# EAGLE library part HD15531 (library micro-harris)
MICROCONTROLLER/MEMORY DEVICE
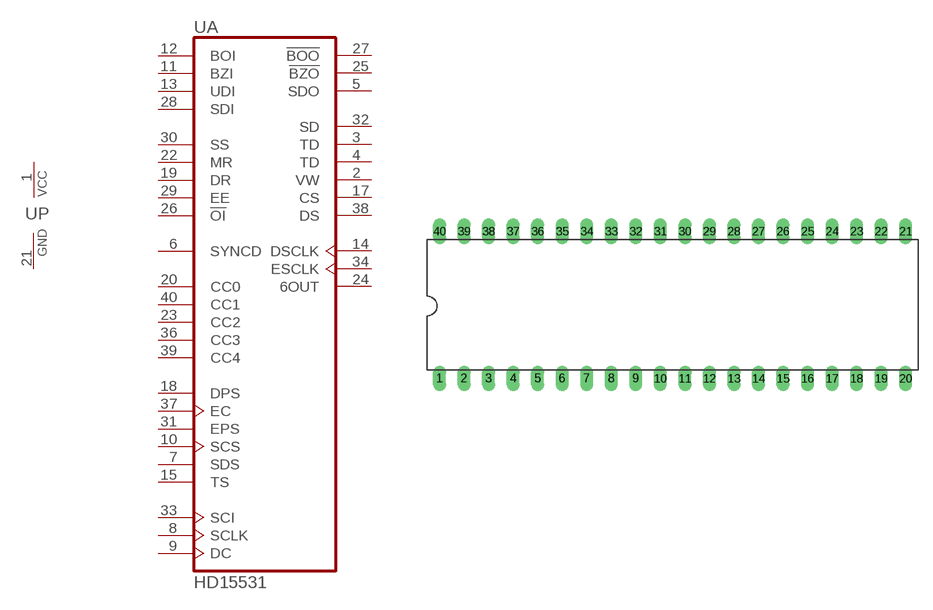
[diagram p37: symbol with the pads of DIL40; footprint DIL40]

Designator prefix U; gates A=HD15531 P=PWRN

## HD15531 (OC_FARNELL: unknown; OC_NEWARK: unknown)  [DIL40]
1  P:VCC  pwr
2  A:VW  out
3  A:TD  out
4  A:TD  out
5  A:SDO  out
6  A:SYNCD  in
7  A:SDS  in
8  A:SCLK  in
9  A:DC  in
10  A:SCS  in
11  A:BZI  in
12  A:BOI  in
13  A:UDI  in
14  A:DSCLK  out
15  A:TS  in
17  A:CS  out
18  A:DPS  in
19  A:DR  in
20  A:CC0  in
21  P:GND  pwr
22  A:MR  in
23  A:CC2  in
24  A:6OUT  out
25  A:!BZO  out
26  A:!OI  in
27  A:!BOO  out
28  A:SDI  in
29  A:EE  in
30  A:SS  in
31  A:EPS  in
32  A:SD  out
33  A:SCI  in
34  A:ESCLK  out
36  A:CC3  in
37  A:EC  in
38  A:DS  out
39  A:CC4  in
40  A:CC1  in

## Footprint DIL40 (pad centres in mm)
Dual In Line Package
drill 0.813 long: 1 -24.13,-7.62; 2 -21.59,-7.62; 3 -19.05,-7.62; 4 -16.51,-7.62; 5 -13.97,-7.62; 6 -11.43,-7.62; 7 -8.89,-7.62; 8 -6.35,-7.62; 9 -3.81,-7.62; 10 -1.27,-7.62; 11 1.27,-7.62; 12 3.81,-7.62; 13 6.35,-7.62; 14 8.89,-7.62; 15 11.43,-7.62; 16 13.97,-7.62; 17 16.51,-7.62; 18 19.05,-7.62; 19 21.59,-7.62; 20 24.13,-7.62; 21 24.13,7.62; 22 21.59,7.62; 23 19.05,7.62; 24 16.51,7.62; 25 13.97,7.62; 26 11.43,7.62; 27 8.89,7.62; 28 6.35,7.62; 29 3.81,7.62; 30 1.27,7.62; 31 -1.27,7.62; 32 -3.81,7.62; 33 -6.35,7.62; 34 -8.89,7.62; 35 -11.43,7.62; 36 -13.97,7.62; 37 -16.51,7.62; 38 -19.05,7.62; 39 -21.59,7.62; 40 -24.13,7.62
